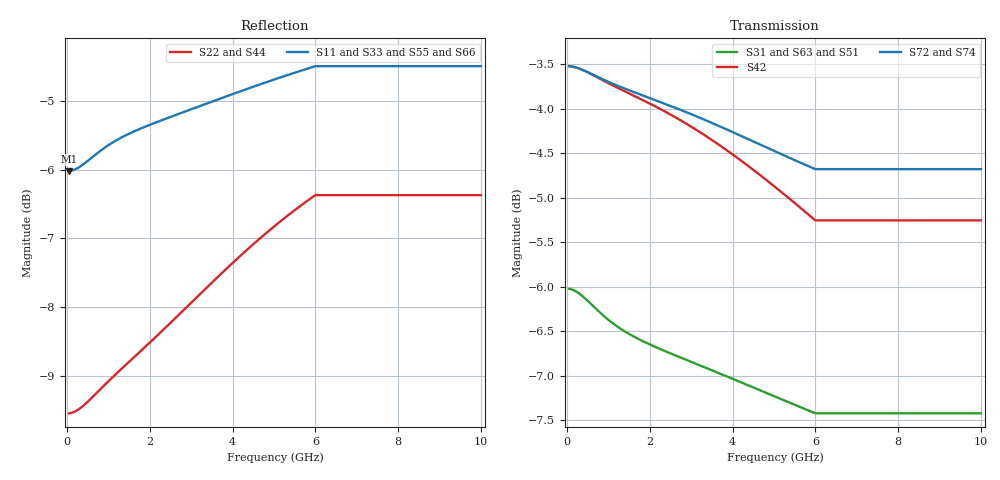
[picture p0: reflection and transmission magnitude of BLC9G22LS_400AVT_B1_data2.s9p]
! Created Mon Aug  3 12:27:02 2015
# ghz S ma R 50
! 9 Port Network Data from SP1.SP block
! freq  magS11  angS11  magS12  angS12  magS13  angS13  magS14  angS14
!  magS15  angS15  magS16  angS16  magS17  angS17  magS18  angS18
!  magS19  angS19
!  magS21  angS21  magS22  angS22  magS23  angS23
!  magS24  angS24  magS25  angS25  magS26  angS26  magS27  angS27
!  magS28  angS28  magS29  angS29
!  magS31  angS31  magS32  angS32
!  magS33  angS33  magS34  angS34  magS35  angS35  magS36  angS36
!  magS37  angS37  magS38  angS38  magS39  angS39
!  magS41  angS41
!  magS42  angS42  magS43  angS43  magS44  angS44  magS45  angS45
!  magS46  angS46  magS47  angS47  magS48  angS48  magS49  angS49
!  magS51  angS51  magS52  angS52  magS53  angS53  magS54  angS54
!  magS55  angS55  magS56  angS56  magS57  angS57  magS58  angS58
!  magS59  angS59
!  magS61  angS61  magS62  angS62  magS63  angS63
!  magS64  angS64  magS65  angS65  magS66  angS66  magS67  angS67
!  magS68  angS68  magS69  angS69
!  magS71  angS71  magS72  angS72
!  magS73  angS73  magS74  angS74  magS75  angS75  magS76  angS76
!  magS77  angS77  magS78  angS78  magS79  angS79
!  magS81  angS81
!  magS82  angS82  magS83  angS83  magS84  angS84  magS85  angS85
!  magS86  angS86  magS87  angS87  magS88  angS88  magS89  angS89
!  magS91  angS91  magS92  angS92  magS93  angS93  magS94  angS94
!  magS95  angS95  magS96  angS96  magS97  angS97  magS98  angS98
!  magS99  angS99
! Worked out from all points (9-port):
!   200 points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, 50 MHz to 10 GHz, reference 50 ohm
!   strongest paths, dB at 50 MHz, 2.55 GHz, 5.05 GHz, 7.55 GHz, 10 GHz:
!     S72: -3.5, -4.0, -4.5, -4.7, -4.7
!     S74: -3.5, -4.0, -4.6, -4.9, -4.9
!     S42: -3.5, -4.1, -4.9, -5.3, -5.3
!     S31: -6.0, -6.8, -7.2, -7.4, -7.4
!     S63: -6.0, -6.8, -7.3, -7.5, -7.5
!     S51: -6.0, -6.8, -7.4, -7.6, -7.6
!   lowest |S11| = -6.0 dB at 50 MHz (marker M1), VSWR 3.00, Z = 16.7 - j0.0434 ohm
!   |S11| at or under -10 dB: nowhere
